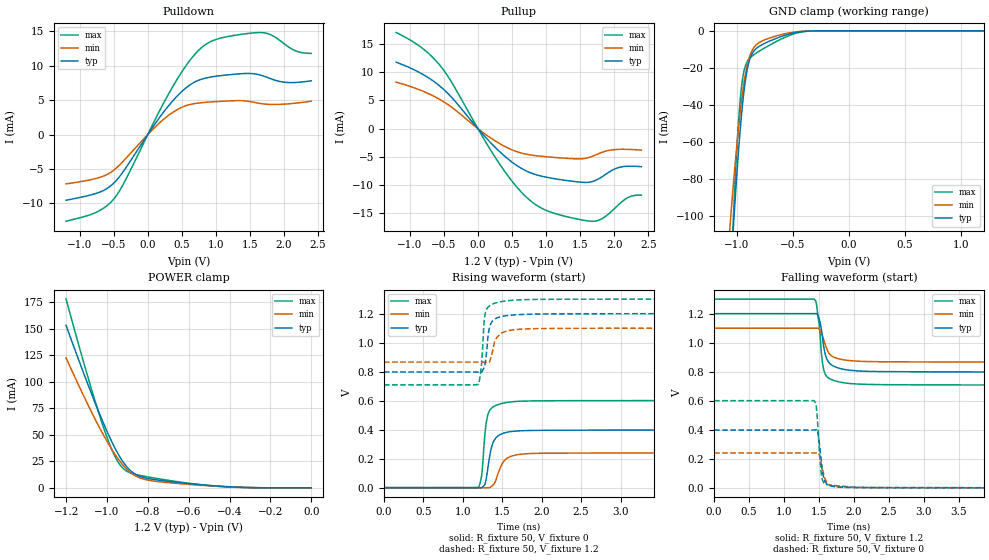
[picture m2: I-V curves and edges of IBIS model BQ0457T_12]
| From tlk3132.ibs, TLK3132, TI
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[Model]   BQ0457T_12
Model_type  I/O
Vinl=0.36
Vinh=0.84
Enable   Active-Low
Vref =   0
Rref =   500
Cref =   5p
Vmeas =   0.6
| variable   typ   min   max
C_comp   1.31pF   1.11pF   1.53pF
| C_pullup   1.34pF   1.08pF   1.71pF
| C_pulldown   1.23pF   0.95pF   1.81pF
| C_tri-state   1.31pF   1.11pF   1.53pF
[Temperature Range]   40   100   -40
| Ambient temperature   25   85   -40
[Voltage range]   1.2   1.1   1.3
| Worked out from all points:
|   slope of the pulldown table from 0 to 0.18 V, typ, clamps not added: 70.1 ohm
|   slope of the pullup table from 0 to 0.18 V, typ, clamps not added: 74.6 ohm
|   GND clamp passes 1 mA (typ) near -0.48 V on its own axis
|   POWER clamp passes 1 mA (typ) near -0.40 V on its own axis
|   rising waveform, R_fixture 50, V_fixture 0: 20-80 % time 87.9ps typ, 122ps min, 62.4ps max; typ from 0 V to 0.398 V
|   falling waveform, R_fixture 50, V_fixture 1.2: 20-80 % time 98.8ps typ, 127ps min, 76ps max; typ from 1.2 V to 0.797 V
|   rising waveform, R_fixture 50, V_fixture 1.2: 20-80 % time 58.2ps typ, 96.1ps min, 46.1ps max; typ from 0.797 V to 1.2 V
|   falling waveform, R_fixture 50, V_fixture 0: 20-80 % time 60.3ps typ, 78.5ps min, 52.5ps max; typ from 0.398 V to 0 V
[GND Clamp]
| BQ0457T_12
|   Voltage   I(typ)   I(min)   I(max)
-1.2V     -312.6mA   -232.8mA   -401.4mA
-1.06V    -139.1mA   -106.9mA   -146.3mA
-1.03V    -108.1mA   -84.21mA   -103.1mA
-1.025V   -103.1mA   -80.61mA   -96.5mA
-985mV    -67.08mA   -54.08mA   -51.42mA
-965mV    -51.73mA   -42.7mA    -35.76mA
-945mV    -38.72mA   -32.88mA   -25.47mA
-920mV    -26.28mA   -23.11mA   -18.72mA
-890mV    -16.99mA   -15.1mA    -15.28mA
-810mV    -8.852mA   -6.822mA   -11.46mA
-375mV    -179.4uA   -116.2uA   -266.1uA
1.2V      163.9nA    3.927uA    4.182nA
[POWER Clamp]
| BQ0457T_12
|   Voltage   I(typ)   I(min)   I(max)
-1.2V     153.1mA    122.4mA    177.7mA
-1.09V    95.84mA    77.15mA    102.3mA
-1.01V    57.77mA    47.38mA    53.15mA
-980mV    45mA       37.45mA    37.84mA
-955mV    35.39mA    29.97mA    27.53mA
-935mV    28.6mA     24.64mA    21.44mA
-910mV    21.54mA    18.96mA    16.63mA
-880mV    15.44mA    13.77mA    13.73mA
-845mV    11.34mA    9.892mA    11.97mA
-720mV    6.595mA    5.26mA     7.742mA
-415mV    1.184mA    1.064mA    938.7uA
-3.398fV  163.9nA    111.1nA    176.7nA
[Pulldown]
| BQ0457T_12
|   Voltage   I(typ)   I(min)   I(max)
-1.2V     -9.542mA   -7.162mA   -12.6mA
-760mV    -8.552mA   -6.381mA   -11.31mA
-485mV    -6.915mA   -5.06mA    -9.187mA
-340mV    -5.087mA   -3.66mA    -6.841mA
360mV     4.807mA    3.169mA    6.837mA
625mV     7.24mA     4.366mA    10.84mA
845mV     8.178mA    4.666mA    13.04mA
1.14V     8.621mA    4.849mA    14.15mA
1.685V    8.529mA    4.457mA    14.78mA
2.015V    7.579mA    4.416mA    13.08mA
2.2V      7.57mA     4.584mA    12.04mA
2.4V      7.794mA    4.834mA    11.77mA
[Pullup]
| BQ0457T_12
|   Voltage   I(typ)   I(min)   I(max)
-1.2V     11.78mA    8.231mA    17.03mA
-830mV    9.762mA    6.746mA    14.38mA
-555mV    7.5mA      5.139mA    11.18mA
350mV     -4.421mA   -2.867mA   -6.835mA
615mV     -6.874mA   -4.25mA    -10.96mA
855mV     -8.175mA   -4.8mA     -13.54mA
1.195V    -9.01mA    -5.173mA   -15.28mA
1.71V     -9.258mA   -4.763mA   -16.41mA
1.855V    -8.281mA   -4.061mA   -15.71mA
2.06V     -6.916mA   -3.675mA   -13.55mA
2.22V     -6.657mA   -3.683mA   -12.11mA
2.4V      -6.746mA   -3.809mA   -11.79mA
[Ramp]
| BQ0457T_12
| variable   typ   min   max
dV/dt_r   0.24/9.58E-11   0.14/1.25E-10   0.36/6.56E-11
dV/dt_f   0.24/1.03E-10   0.14/1.32E-10   0.35/7.86E-11
R_load = 50
[Rising Waveform]
| BQ0457T_12
R_fixture =   50
C_fixture =   0
L_fixture =   0
V_fixture =   0
V_fixture_min = 0
V_fixture_max = 0
|   Time   V(typ)   V(min)   V(max)
0s        25.03uV    24.05uV    27.57uV
1.2ns     -401.6uV   24.71uV    2.32mV
1.24ns    55.94uV    8.703uV    85.17mV
1.28ns    22.2mV     -395.1uV   363.1mV
1.305ns   87.28mV    -763.4uV   470.6mV
1.34ns    212mV      125.8uV    531.4mV
1.43ns    349.2mV    68.97mV    569.5mV
1.545ns   379.9mV    195.9mV    586.6mV
1.74ns    392.3mV    230.6mV    596.2mV
30.51ns   398.2mV    240.3mV    600.5mV
[Falling Waveform]
| BQ0457T_12
R_fixture =   50
C_fixture =   0
L_fixture =   0
V_fixture =   1.2
V_fixture_min = 1.1
V_fixture_max = 1.3
|   Time   V(typ)   V(min)   V(max)
0s        1.2V       1.1V       1.3V
1.43ns    1.2V       1.1V       1.3V
1.46ns    1.201V     1.1V       1.28V
1.505ns   1.162V     1.093V     1.121V
1.55ns    1.046V     1.049V     868.8mV
1.6ns     905.7mV    975.7mV    774.6mV
1.65ns    860.3mV    924mV      753.3mV
1.73ns    834.3mV    897mV      737.5mV
2.1ns     804.4mV    871.7mV    714.2mV
30.51ns   797.5mV    865.9mV    708.5mV
[Rising Waveform]
| BQ0457T_12
R_fixture =   50
C_fixture =   0
L_fixture =   0
V_fixture =   1.2
V_fixture_min = 1.1
V_fixture_max = 1.3
|   Time   V(typ)   V(min)   V(max)
0s        797.5mV    865.9mV    708.5mV
1.2ns     796.4mV    865.9mV    711.9mV
1.24ns    797.2mV    865.8mV    867.5mV
1.275ns   835.4mV    864.9mV    1.168V
1.305ns   953.9mV    863.9mV    1.234V
1.33ns    1.082V     862.7mV    1.249V
1.38ns    1.151V     946.5mV    1.267V
1.485ns   1.179V     1.063V     1.282V
1.765ns   1.194V     1.093V     1.296V
30.51ns   1.2V       1.1V       1.3V
[Falling Waveform]
| BQ0457T_12
R_fixture =   50
C_fixture =   0
L_fixture =   0
V_fixture =   0
V_fixture_min = 0
V_fixture_max = 0
|   Time   V(typ)   V(min)   V(max)
0s        398.2mV    240.4mV    600.5mV
1.43ns    398.4mV    240.4mV    600.8mV
1.46ns    400.2mV    240.8mV    572mV
1.485ns   379.2mV    241.2mV    424.3mV
1.53ns    206.5mV    175.6mV    117.9mV
1.565ns   78.27mV    101.9mV    38.74mV
1.6ns     34.54mV    49.4mV     24.2mV
1.655ns   15.68mV    20.86mV    20.19mV
2.045ns   2.586mV    2.027mV    3.89mV
30.51ns   30.85uV    26.85uV    33.86uV
